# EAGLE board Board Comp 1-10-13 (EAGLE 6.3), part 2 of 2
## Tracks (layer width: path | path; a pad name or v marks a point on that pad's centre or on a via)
3.3V1  (via drill 0.61)
  Top 0.406: v91.72,21.72 107.04,21.72 108.41,20.34 109.17,20.34 SV1.6
  Bottom 0.406: 317CAP8.1 86.16,25.38 84.56,25.38 81.97,22.78 R7.1 81.81,22.55 81.81,21.49 80.52,20.19 80.52,18.21 80.82,17.91 84.63,17.91 88.75,22.02 IC4.4 88.9,22.1 89.28,21.72 v91.72,21.72
3.3V1_EN  (via drill 0.61)
  Top 0.406: v113.36,4.95 114.5,4.95 116.79,2.67 S1.19 | v101.62,6.4 98.65,6.4 98.27,6.02 96.37,6.02 v88.59,13.79
  Bottom 0.406: 317CAP3.1 93.17,56.46 93.17,52.2 91.95,50.98 80.82,50.98 79.15,49.3 79.15,16.76 80.82,15.09 85.7,15.09 86.54,15.93 IC4.3 86.61,15.77 v88.59,13.79 | v113.36,4.95 108.94,4.95 107.49,6.4 v101.62,6.4
3.3V1_EN1  (via drill 0.61)
  Top 0.406: v113.36,82.42 114.5,82.42 116.79,80.14 S2.19 | v101.62,83.87 98.65,83.87 98.27,83.49 96.37,83.49 v88.59,91.26
  Bottom 0.406: 317CAP1.1 93.17,133.93 93.17,129.67 91.95,128.45 80.82,128.45 79.15,126.77 79.15,94.23 80.82,92.56 85.7,92.56 86.54,93.4 IC3.3 86.61,93.24 v88.59,91.26 | v113.36,82.42 108.94,82.42 107.49,83.87 v101.62,83.87
3.3V2  (via drill 0.61)
  Top 0.406: v105.36,43.05 96.29,52.12 v91.72,52.12
  Bottom 0.406: 317CAP10.1 86.23,56.46 86.23,55.32 88.9,52.65 IC5.4 | R9.1 81.97,53.26 88.06,53.26 IC5.4 | v105.36,43.05 105.36,27.51 106.66,26.21 106.66,20.34 SV1.4 | v91.72,52.12 89.43,52.12 89.05,52.5 IC5.4
3.3V2_EN  (via drill 0.61)
  Top 0.406: v107.87,9.07 114.28,2.67 S1.18 | v97.05,33.3 v105.36,24.99
  Bottom 0.406: 92.63,43.13 91.34,43.13 89.97,41.76 88.06,41.76 87.53,42.29 87.53,45.49 IC5.3 | 92.63,43.13 93.78,43.13 317CAP9.1 | v107.87,9.07 107.87,14.86 105.36,17.37 v105.36,24.99 | v97.05,33.3 97.05,33.91 92.63,38.33 92.63,43.13
3.3V2_EN1  (via drill 0.61)
  Top 0.406: v107.87,86.54 114.28,80.14 S2.18 | v97.05,110.77 v105.36,102.46
  Bottom 0.406: 92.63,120.6 91.34,120.6 89.97,119.23 88.06,119.23 87.53,119.76 87.53,122.96 IC7.3 | 92.63,120.6 93.78,120.6 317CAP4.1 | v107.87,86.54 107.87,92.33 105.36,94.84 v105.36,102.46 | v97.05,110.77 97.05,111.38 92.63,115.8 92.63,120.6
3.3V3  (via drill 0.61)
  Top 0.406: v98.73,20.73 99.11,20.34 104.14,20.34 SV1.2
  Bottom 0.406: IC6.4 86.23,42.6 86.23,43.13 317CAP12.1 | IC6.4 | R11.1 81.97,39.93 88.67,39.93 IC6.4 | v98.73,20.73 98.73,30.02 88.98,39.78 IC6.4
3.3V3_EN  (via drill 0.61)
  Top 0.406: S1.17 111.76,3.12 105.36,9.53 100.79,9.53 90.73,19.58 90.73,24.23 v91.34,24.84
  Bottom 0.406: 93.17,26.52 93.17,27.66 92.33,28.5 92.33,35.05 92.02,35.36 88.14,35.36 86.54,33.76 IC6.3 | 93.17,26.52 93.17,25.45 317CAP11.1 | v91.34,24.84 93.02,26.52 93.17,26.52
3.3V3_EN1  (via drill 0.61)
  Top 0.406: S2.17 111.76,80.59 105.36,87 100.79,87 90.73,97.05 90.73,101.7 v91.34,102.31
  Bottom 0.406: 93.17,103.99 93.17,105.13 92.33,105.97 92.33,112.52 92.02,112.83 88.14,112.83 86.54,111.23 IC8.3 | 93.17,103.99 93.17,102.92 317CAP6.1 | v91.34,102.31 93.02,103.99 93.17,103.99
3.3V4  (via drill 0.61)
  Top 0.406: v98.73,98.2 99.11,97.81 104.14,97.81 SV5.2
  Bottom 0.406: IC8.4 86.23,120.07 86.23,120.6 317CAP7.1 | IC8.4 | R13.1 81.97,117.4 88.67,117.4 IC8.4 | v98.73,98.2 98.73,107.49 88.98,117.25 IC8.4
3.3V5  (via drill 0.61)
  Top 0.406: v91.72,99.19 107.04,99.19 108.41,97.81 109.17,97.81 SV5.6
  Bottom 0.406: 317CAP2.1 86.16,102.84 84.56,102.84 81.97,100.25 R3.1 81.81,100.03 81.81,98.96 80.52,97.66 80.52,95.68 80.82,95.38 84.63,95.38 88.75,99.49 IC3.4 88.9,99.57 89.28,99.19 v91.72,99.19
3.3V6  (via drill 0.61)
  Top 0.406: v105.36,120.52 96.29,129.59 v91.72,129.59
  Bottom 0.406: 317CAP5.1 86.23,133.93 86.23,132.79 88.9,130.12 IC7.4 | R5.1 81.97,130.73 88.06,130.73 IC7.4 | v105.36,120.52 105.36,104.98 106.66,103.68 106.66,97.81 SV5.4 | v91.72,129.59 89.43,129.59 89.05,129.97 IC7.4
5V1  (via drill 0.61)
  Top 0.406: v123.19,26.67 127.46,26.67 139.88,39.09 v139.88,41.99
  Bottom 0.406: C4.1 148.41,52.12 148.41,52.35 146.43,54.33 140.56,54.33 140.34,54.1 140.34,47.47 141.17,46.63 141.17,43.51 PWR_1.2 141.17,43.28 v139.88,41.99 | v123.19,26.67 SV1.12
5V1_EN  (via drill 0.61)
  Top 0.406: v126.01,4.8 124.48,3.28 124.48,2.67 S1.22 | v130.66,4.95 130.66,8.84 131.34,9.53 v131.34,21.41
  Bottom 0.406: C3.1 148.41,44.42 147.5,43.51 145.82,43.51 PWR_1.1 145.59,43.43 143.69,43.43 131.34,31.09 v131.34,21.41 | v126.01,4.8 130.5,4.8 v130.66,4.95
5V1_EN1  (via drill 0.61)
  Top 0.406: v126.01,82.27 124.48,80.75 124.48,80.14 S2.22 | v130.66,82.42 130.66,86.31 131.34,87 v131.34,98.88
  Bottom 0.406: C9.1 148.41,121.89 147.5,120.98 145.82,120.98 PWR_4.1 145.59,120.9 143.69,120.9 131.34,108.56 v131.34,98.88 | v126.01,82.27 130.5,82.27 v130.66,82.42
5V2  (via drill 0.61)
  Top 0.406: v147.8,36.12 v143.84,32.16 | v134.85,23.09 117.86,23.09 115.11,20.34 114.35,20.34 SV1.10
  Bottom 0.406: v143.84,32.16 141.25,29.57 PWR_2.2 141.1,29.34 v134.85,23.09 | v147.8,36.12 147.8,37.49 148.41,38.1 C6.1
5V2_EN  (via drill 0.61)
  Top 0.406: v124.56,4.88 124.18,4.88 121.97,2.67 S1.21 | v132.1,3.66 135.15,3.66 146.89,15.39 v146.89,27.81
  Bottom 0.406: 146.77,31.2 147.42,31.85 149.86,31.85 151.23,30.48 C5.1 | 146.77,31.2 145.82,30.25 145.82,29.57 PWR_2.1 | v124.56,4.88 125.78,3.66 v132.1,3.66 | v146.89,27.81 146.89,31.09 146.77,31.2
5V2_EN1  (via drill 0.61)
  Top 0.406: v124.56,82.35 124.18,82.35 121.97,80.14 S2.21 | v132.1,81.13 135.15,81.13 146.89,92.86 v146.89,105.28
  Bottom 0.406: 146.77,108.67 147.42,109.32 149.86,109.32 151.23,107.95 C11.1 | 146.77,108.67 145.82,107.72 145.82,107.04 PWR_5.1 | v124.56,82.35 125.78,81.13 v132.1,81.13 | v146.89,105.28 146.89,108.56 146.77,108.67
5V3  (via drill 0.61)
  Top 0.406: v141.17,18.14 135.23,24.08 116.33,24.08 112.6,20.34 111.76,20.34 SV1.8
  Bottom 0.406: C7.1 148.41,24.08 148.41,21.26 142.7,15.54 141.25,15.54 PWR_3.2 141.17,15.7 v141.17,18.14
5V3_EN  (via drill 0.61)
  Top 0.406: v125.32,5.94 122.81,5.94 119.53,2.67 119.38,2.67 S1.20 | v133.02,5.94 136.07,5.94 v144.37,14.25
  Bottom 0.406: C8.1 148.41,16.46 147.5,15.54 145.82,15.54 PWR_3.1 145.59,15.47 v144.37,14.25 | v133.02,5.94 v125.32,5.94
5V3_EN1  (via drill 0.61)
  Top 0.406: v125.32,83.41 122.81,83.41 119.53,80.14 119.38,80.14 S2.20 | v133.02,83.41 136.07,83.41 v144.37,91.72
  Bottom 0.406: C14.1 148.41,93.93 147.5,93.02 145.82,93.02 PWR_6.1 145.59,92.94 v144.37,91.72 | v133.02,83.41 v125.32,83.41
5V4  (via drill 0.61)
  Top 0.406: v141.17,95.61 135.23,101.55 116.33,101.55 112.6,97.81 111.76,97.81 SV5.8
  Bottom 0.406: C13.1 148.41,101.55 148.41,98.73 142.7,93.02 141.25,93.02 PWR_6.2 141.17,93.17 v141.17,95.61
5V5  (via drill 0.61)
  Top 0.406: v147.8,113.59 v143.84,109.63 | v134.85,100.56 117.86,100.56 115.11,97.81 114.35,97.81 SV5.10
  Bottom 0.406: v143.84,109.63 141.25,107.04 PWR_5.2 141.1,106.81 v134.85,100.56 | v147.8,113.59 147.8,114.96 148.41,115.57 C12.1
5V6  (via drill 0.61)
  Top 0.406: v123.19,104.14 127.46,104.14 139.88,116.56 v139.88,119.46
  Bottom 0.406: C10.1 148.41,129.59 148.41,129.82 146.43,131.8 140.56,131.8 140.34,131.57 140.34,124.94 141.17,124.1 141.17,120.98 PWR_4.2 141.17,120.75 v139.88,119.46 | v123.19,104.14 SV5.12
5V7
  Top 0.406: UP_TIME1.3 170.18,61.98 168.66,63.5 168.66,89.15 IC11.8 IC11.4 168.91,104.14 IC12.3
12V  (via drill 0.61)
  Top 0.406: 198.37,139.19 198.37,139.32 201.93,142.88 203.07,142.88 204.47,141.48 POWER.2 | 198.37,139.19 198.37,137.16 C1.1 | J2.1 161.29,138.05 162.81,136.53 163.7,136.53 167.89,140.72 167.89,144.91 U$2.1 167.89,145.03 167,145.92 167,148.46 167.77,149.22 170.05,149.22 173.1,146.18 178.56,146.18 | 178.56,146.18 182.25,146.18 U$4.8 | IC1.3 182.88,131.7 184.02,132.84 v184.02,133.73 | 178.56,146.18 v178.56,139.19 | v196.34,139.19 198.37,139.19
  Bottom 0.406: v184.02,133.73 v178.56,139.19 v196.34,139.19
12V1  (via drill 0.61)
  Top 0.406: 208.79,100.58 208.66,100.58 205.1,104.14 205.1,105.28 206.5,106.68 POWER1.2 | 208.79,100.58 210.82,100.58 C2.1 | J1.1 209.93,63.5 211.46,65.02 211.46,65.91 207.26,70.1 203.07,70.1 U$6.1 202.95,70.1 202.06,69.22 199.52,69.22 198.75,69.98 198.75,72.26 201.8,75.31 201.8,80.77 | 201.8,80.77 201.8,84.45 U$8.8 | IC2.3 216.28,85.09 215.14,86.23 v214.25,86.23 | 201.8,80.77 v208.79,80.77 | v208.79,98.55 208.79,100.58
  Bottom 0.406: v214.25,86.23 v208.79,80.77 v208.79,98.55
12V1_EN
  Top 0.406: S1.24 129.59,2.67 129.59,8.76 130.66,9.83 130.66,18.44 127.53,21.57 123.19,21.57 121.97,20.34 SV1.16
12V1_EN1
  Top 0.406: S2.24 129.59,80.14 129.59,86.23 130.66,87.3 130.66,95.91 127.53,99.03 123.19,99.03 121.97,97.81 SV5.16
12V2
  Top 1.27: SV1.18 124.48,20.34 127,20.34 SV1.20 127.38,19.81 128.68,18.52 128.68,11.2 | S1.11 101.62,11.2 S1.12 | S1.11 | S1.11 106.66,11.2 | 106.66,11.2 S1.10 | 106.66,11.2 109.17,11.2 S1.9 109.86,11.2 S1.8 | S1.8 | S1.8 114.28,11.2 | 114.28,11.2 S1.7 | 114.28,11.2 116.79,11.2 S1.6 117.47,11.2 S1.5 | S1.5 | S1.5 121.89,11.2 | 121.89,11.2 S1.4 | 121.89,11.2 124.41,11.2 S1.3 125.09,11.2 S1.2 | S1.2 | S1.2 128.68,11.2 | 128.68,11.2 129.51,11.2 S1.1
  Bottom 1.27: 12V_INPUT.1 117.32,62.87 128.68,51.51 128.68,22.02 127,20.34 SV1.20
12V2_EN  (via drill 0.61)
  Top 0.406: v127,8.91 S1.23
  Bottom 0.406: v127,8.91 127,10.97 120.6,17.37 120.6,19.05 119.38,20.27 SV1.14
12V2_EN1  (via drill 0.61)
  Top 0.406: v127,86.39 S2.23
  Bottom 0.406: v127,86.39 127,88.44 120.6,94.84 120.6,96.52 119.38,97.74 SV5.14
12V3
  Top 1.27: SV5.18 124.48,97.81 127,97.81 SV5.20 127.38,97.28 128.68,95.99 128.68,88.67 | S2.11 101.62,88.67 S2.12 | S2.11 | S2.11 106.66,88.67 | 106.66,88.67 S2.10 | 106.66,88.67 109.17,88.67 S2.9 109.86,88.67 S2.8 | S2.8 | S2.8 114.28,88.67 | 114.28,88.67 S2.7 | 114.28,88.67 116.79,88.67 S2.6 117.47,88.67 S2.5 | S2.5 | S2.5 121.89,88.67 | 121.89,88.67 S2.4 | 121.89,88.67 124.41,88.67 S2.3 125.09,88.67 S2.2 | S2.2 | S2.2 128.68,88.67 | 128.68,88.67 129.51,88.67 S2.1
  Bottom 1.27: 12V_INPUT1.1 117.32,140.34 128.68,128.98 128.68,99.49 127,97.81 SV5.20
12V4
  Top 2.54: 72.39,100.84 R15.2 R16.2 67.31,100.84 66.24,101.55 64.29,103.5 55.78,103.5 53.82,105.46 53.82,122.15 54.71,123.04 | 54.71,123.04 54.86,122.89 56.84,122.89 D3.C | 54.71,123.04 52.93,124.82 45.59,124.82 44.35,123.57 44.35,123.55 44.12,123.32 44.12,123.14 43.99,123.01 43.99,122.89 43.28,122.17 43.28,122 41.94,120.65 K2.P1
12V5
  Top 2.54: 72.39,23.37 R21.2 R22.2 67.31,23.37 66.24,24.08 64.29,26.04 55.78,26.04 53.82,27.99 53.82,44.68 54.71,45.57 | 54.71,45.57 54.86,45.41 56.84,45.41 D1.C | 54.71,45.57 52.93,47.35 45.59,47.35 44.35,46.1 44.35,46.08 44.12,45.85 44.12,45.67 43.99,45.54 43.99,45.41 43.28,44.7 43.28,44.53 41.94,43.18 K4.P1
12V6  (via drill 0.61)
  Top 0.406: 208.79,43.43 208.66,43.43 205.1,46.99 205.1,48.13 206.5,49.53 POWER4.2 | 208.79,43.43 210.82,43.43 C21.1 | J3.1 209.93,6.35 211.46,7.87 211.46,8.76 207.26,12.95 203.07,12.95 U$12.1 202.95,12.95 202.06,12.06 199.52,12.06 198.75,12.83 198.75,15.11 201.8,18.16 201.8,23.62 | 201.8,23.62 201.8,27.3 U$14.8 | IC13.3 216.28,27.94 215.14,29.08 v214.25,29.08 | 201.8,23.62 v208.79,23.62 | v208.79,41.4 208.79,43.43
  Bottom 0.406: v214.25,29.08 v208.79,23.62 v208.79,41.4
12V7  (via drill 0.61)
  Top 0.406: 235.46,100.58 235.33,100.58 231.78,104.14 231.78,105.28 233.17,106.68 POWER5.2 | 235.46,100.58 237.49,100.58 C15.1 | J4.1 236.6,63.5 238.12,65.02 238.12,65.91 233.93,70.1 229.74,70.1 U$16.1 229.62,70.1 228.73,69.22 226.19,69.22 225.43,69.98 225.43,72.26 228.47,75.31 228.47,80.77 | 228.47,80.77 228.47,84.45 U$18.8 | IC9.3 242.95,85.09 241.81,86.23 v240.92,86.23 | 228.47,80.77 v235.46,80.77 | v235.46,98.55 235.46,100.58
  Bottom 0.406: v240.92,86.23 v235.46,80.77 v235.46,98.55
12V8  (via drill 0.61)
  Top 0.406: 235.46,43.43 235.33,43.43 231.78,46.99 231.78,48.13 233.17,49.53 POWER6.2 | 235.46,43.43 237.49,43.43 C16.1 | J5.1 236.6,6.35 238.12,7.87 238.12,8.76 233.93,12.95 229.74,12.95 U$20.1 229.62,12.95 228.73,12.06 226.19,12.06 225.43,12.83 225.43,15.11 228.47,18.16 228.47,23.62 | 228.47,23.62 228.47,27.3 U$22.8 | IC10.3 242.95,27.94 241.81,29.08 v240.92,29.08 | 228.47,23.62 v235.46,23.62 | v235.46,41.4 235.46,43.43
  Bottom 0.406: v240.92,29.08 v235.46,23.62 v235.46,41.4
12V_PRE
  Top 2.54: D3.A 65.02,107.95 69.47,112.39 POWER2.2
12V_PRE1
  Top 2.54: D1.A 65.02,30.48 69.47,34.92 POWER3.2
24V1
  Top 0.406: IC12.1 177.8,106.68 C20.+ | LED9.A 162.69,35.56 173.99,24.26 X2.3
  Bottom 0.406: C20.+ 184.15,106.81 186.94,104.01 186.94,62.48 LED9.A
DIR
  Top 0.406: R17.2 53.34,146.51 51.61,148.23 51.05,148.23 IO.2
DIR1
  Top 0.406: R23.2 53.34,69.04 51.61,70.76 51.05,70.76 IO1.2
GND
  pour Top: 156.21,152.4 156.21,129.54 209.55,129.54 209.55,152.4
  pour Bottom: 156.21,152.4 156.21,129.54 209.55,129.54 209.55,152.4
GND1
  pour Top: 195.58,58.42 218.44,58.42 218.44,111.76 195.58,111.76
  pour Bottom: 195.58,58.42 218.44,58.42 218.44,111.76 195.58,111.76
GND2  (via drill 0.61)
  Top 0.406: U$9.9 137.52,67.28 137.52,62.26 U$9.7 137.36,62.18 136.6,62.18 134.43,60.01 | SV4.1 104.14,48.31 106.66,48.31 SV4.3 106.88,48.23 109.17,48.23 SV4.5 109.4,48.31 111.76,48.31 SV4.7 111.91,48.31 114.28,48.31 SV4.9 114.5,48.23 116.79,48.23 SV4.11 117.02,48.31 119.38,48.31 SV4.13 119.53,48.31 121.89,48.31 SV4.15 122.12,48.23 124.41,48.23 SV4.17 124.64,48.31 125.78,48.31 | 125.78,48.31 127,48.31 SV4.19 127.08,48.08 127.08,42.29 128.22,41.15 128.22,39.4 127.08,38.25 SV3.19 SV3.17 SV3.15 SV3.13 SV3.11 SV3.9 SV3.7 SV3.5 SV3.3 SV3.1 104.06,37.95 104.06,32.16 102.92,31.01 102.92,29.26 104.06,28.12 SV2.1 104.14,27.96 106.66,27.96 SV2.3 106.81,27.96 109.17,27.96 SV2.5 109.4,27.96 110.54,27.96 | 134.43,60.01 125.78,51.36 125.78,48.31 | SV1.1 104.14,17.83 106.66,17.83 SV1.3 | 110.54,27.96 111.76,27.96 SV2.7 111.91,27.96 114.28,27.96 SV2.9 114.43,27.96 116.79,27.96 SV2.11 117.02,27.96 119.38,27.96 SV2.13 119.53,27.96 121.89,27.96 SV2.15 122.05,27.96 124.41,27.96 SV2.17 124.64,27.96 127,27.96 SV2.19 | SV1.19 127,17.83 124.64,17.83 SV1.17 124.41,17.83 121.97,17.83 SV1.15 121.74,17.83 119.38,17.83 SV1.13 | 110.54,19.05 110.54,27.96 | 110.54,19.05 111.76,17.83 SV1.7 | SV1.5 109.25,17.83 110.39,18.97 110.54,19.05 | 134.43,60.01 v130.89,63.55
  Bottom 0.406: 130.66,63.55 130.66,65.99 V7805_C5.2 130.66,66.22 130.66,69.19 | 130.66,63.55 130.66,61.65 V7805_C6.2 | 130.66,69.19 130.66,70.48 V7805_C4.2 | 130.66,69.19 116.86,69.19 12V_INPUT.2 116.71,69.19 101.78,69.19 TS7800_CON.2 | R12.2 81.89,36.35 81.89,36.5 79.83,38.56 79.83,47.55 81.89,49.61 R10.2 | SV1.3 106.73,17.75 108.94,17.75 SV1.5 | C6.2 151.23,38.1 151.23,44.42 C3.2 | SV1.7 111.76,17.83 114.12,17.83 SV1.9 114.58,17.75 116.79,17.75 SV1.11 117.02,17.83 119.38,17.83 SV1.13 | v130.89,63.55 130.66,63.55
  pour Top: 78.74,74.93 152.4,74.93 152.4,1.27 78.74,1.27
  pour Bottom: 78.74,74.93 152.4,74.93 152.4,1.27 78.74,1.27
GND3  (via drill 0.61)
  Top 0.406: U$10.9 137.52,144.75 137.52,139.72 U$10.7 137.36,139.65 136.6,139.65 134.43,137.48 | SV8.1 104.14,125.78 106.66,125.78 SV8.3 106.88,125.7 109.17,125.7 SV8.5 109.4,125.78 111.76,125.78 SV8.7 111.91,125.78 114.28,125.78 SV8.9 114.5,125.7 116.79,125.7 SV8.11 117.02,125.78 119.38,125.78 SV8.13 119.53,125.78 121.89,125.78 SV8.15 122.12,125.7 124.41,125.7 SV8.17 124.64,125.78 125.78,125.78 | 125.78,125.78 127,125.78 SV8.19 127.08,125.55 127.08,119.76 128.22,118.62 128.22,116.86 127.08,115.72 SV7.19 SV7.17 SV7.15 SV7.13 SV7.11 SV7.9 SV7.7 SV7.5 SV7.3 SV7.1 104.06,115.42 104.06,109.63 102.92,108.48 102.92,106.73 104.06,105.59 SV6.1 104.14,105.44 106.66,105.44 SV6.3 106.81,105.44 109.17,105.44 SV6.5 109.4,105.44 110.54,105.44 | 134.43,137.48 125.78,128.83 125.78,125.78 | SV5.1 104.14,95.3 106.66,95.3 SV5.3 | 110.54,105.44 111.76,105.44 SV6.7 111.91,105.44 114.28,105.44 SV6.9 114.43,105.44 116.79,105.44 SV6.11 117.02,105.44 119.38,105.44 SV6.13 119.53,105.44 121.89,105.44 SV6.15 122.05,105.44 124.41,105.44 SV6.17 124.64,105.44 127,105.44 SV6.19 | SV5.19 127,95.3 124.64,95.3 SV5.17 124.41,95.3 121.97,95.3 SV5.15 121.74,95.3 119.38,95.3 SV5.13 | 110.54,96.52 110.54,105.44 | 110.54,96.52 111.76,95.3 SV5.7 | SV5.5 109.25,95.3 110.39,96.44 110.54,96.52 | 134.43,137.48 v130.89,141.02
  Bottom 0.406: 130.66,141.02 130.66,143.46 V7805_C2.2 130.66,143.69 130.66,146.66 | 130.66,141.02 130.66,139.12 V7805_C3.2 | 130.66,146.66 130.66,147.96 V7805_C1.2 | 130.66,146.66 116.86,146.66 12V_INPUT1.2 116.71,146.66 101.78,146.66 TS7800_CON1.2 | R14.2 81.89,113.82 81.89,113.97 79.83,116.03 79.83,125.02 81.89,127.08 R6.2 | SV5.3 106.73,95.22 108.94,95.22 SV5.5 | C12.2 151.23,115.57 151.23,121.89 C9.2 | SV5.7 111.76,95.3 114.12,95.3 SV5.9 114.58,95.22 116.79,95.22 SV5.11 117.02,95.3 119.38,95.3 SV5.13 | v130.89,141.02 130.66,141.02
  pour Top: 78.74,152.4 152.4,152.4 152.4,78.74 78.74,78.74
  pour Bottom: 78.74,152.4 152.4,152.4 152.4,78.74 78.74,78.74
GND4
  pour Top: 222.25,58.42 245.11,58.42 245.11,111.76 222.25,111.76
  pour Bottom: 222.25,58.42 245.11,58.42 245.11,111.76 222.25,111.76
GND5
  pour Bottom: 156.21,1.27 191.77,1.27 191.77,125.73 156.21,125.73
  pour Top: 156.21,1.27 191.77,1.27 191.77,125.73 156.21,125.73
GND6
  pour Top: 1.27,152.4 74.93,152.4 74.93,78.74 1.27,78.74
  pour Bottom: 1.27,152.4 74.93,152.4 74.93,78.74 1.27,78.74
GND7
  pour Top: 1.27,74.93 74.93,74.93 74.93,1.27 1.27,1.27
  pour Bottom: 1.27,74.93 74.93,74.93 74.93,1.27 1.27,1.27
GND8
  pour Top: 195.58,1.27 218.44,1.27 218.44,54.61 195.58,54.61
  pour Bottom: 195.58,1.27 218.44,1.27 218.44,54.61 195.58,54.61
GND9
  pour Top: 222.25,1.27 245.11,1.27 245.11,54.61 222.25,54.61
  pour Bottom: 222.25,1.27 245.11,1.27 245.11,54.61 222.25,54.61
MOTOR+
  Bottom 2.54: K1.O2 36.96,97.92 38.23,99.19 38.23,99.67 39.22,100.66 39.22,100.71 40.18,101.68 40.31,101.68 40.49,101.85 40.77,101.85 40.89,101.98 41.02,101.98 41.1,101.91 43.31,101.91 43.59,101.62 43.66,101.7 43.71,101.7 44.91,102.89 44.91,103.35 46.91,105.36 46.91,105.41 K1.S1 47.98,106.15 50.11,108.28 50.11,124.28 27.66,146.74 27.66,147.32 OUTPUT.2
MOTOR+1
  Bottom 2.54: K3.O2 36.96,20.45 38.23,21.72 38.23,22.2 39.22,23.19 39.22,23.24 40.18,24.21 40.31,24.21 40.49,24.38 40.77,24.38 40.89,24.51 41.02,24.51 41.1,24.43 43.31,24.43 43.59,24.16 43.66,24.23 43.71,24.23 44.91,25.43 44.91,25.88 46.91,27.89 46.91,27.94 K3.S1 47.98,28.68 50.11,30.81 50.11,46.81 27.66,69.27 27.66,69.85 OUTPUT1.2
MOTOR-
  Top 2.54: K1.S2 46.91,97.92 46.91,97.97 44.91,99.97 44.91,100.43 43.71,101.62 43.66,101.62 43.59,101.7 43.31,101.42 41.1,101.42 41.02,101.35 40.89,101.35 40.77,101.47 40.49,101.47 40.31,101.65 40.18,101.65 39.22,102.62 39.22,102.67 38.23,103.66 38.23,104.14 36.96,105.41 K1.O1 35.89,106.15 34.14,107.9 34.14,133.91 21.31,146.74 OUTPUT.1
MOTOR-1
  Top 2.54: K3.S2 46.91,20.45 46.91,20.5 44.91,22.5 44.91,22.96 43.71,24.16 43.66,24.16 43.59,24.23 43.31,23.95 41.1,23.95 41.02,23.88 40.89,23.88 40.77,24 40.49,24 40.31,24.18 40.18,24.18 39.22,25.15 39.22,25.2 38.23,26.19 38.23,26.67 36.96,27.94 K3.O1 35.89,28.68 34.14,30.43 34.14,56.44 21.31,69.27 OUTPUT1.1
N$1  (via drill 0.61)
  Top 0.406: v189.48,132.08 U$1.1 | v182.75,132.97 181.61,131.83 IC1.2
  Bottom 0.406: v189.48,132.08 183.64,132.08 v182.75,132.97
N$2  (via drill 0.61)
  Top 0.406: v198.37,135.13 198.37,132.08 U$1.2 | v198.37,141.99 200.03,143.64 U$3.1
  Bottom 0.406: v198.37,141.99 v198.37,135.13
N$3  (via drill 0.61)
  Top 0.406: IC1.4 184.15,131.95 v185.29,133.1 | v180.97,138.18 178.05,138.18 171.07,131.19 168.91,131.19 R1.2
  Bottom 0.406: v185.29,133.1 185.29,133.86 v180.97,138.18
N$4
  Top 0.406: U$2.2 169.8,144.91 169.8,139.19 166.24,135.64 R1.3
N$5
  Top 0.406: C1.2 195.33,137.16 195.33,144.4 193.68,146.05 U$3.4 | U$3.4 U$3.2 | J2.2 161.29,143.76 167.51,149.99 189.48,149.99 193.55,145.92 U$3.4
N$6  (via drill 0.61)
  Top 0.406: v215.9,91.69 U$5.1 | v215.01,84.96 216.15,83.82 IC2.2
  Bottom 0.406: v215.9,91.69 215.9,85.85 v215.01,84.96
N$7  (via drill 0.61)
  Top 0.406: IC2.4 216.03,86.36 v214.88,87.5 | v209.8,83.19 209.8,80.26 216.79,73.28 216.79,71.12 R2.2
  Bottom 0.406: v214.88,87.5 214.12,87.5 v209.8,83.19
N$8
  Top 0.406: IC1.5 185.42,131.57 187.58,133.73 188.72,133.73 189.48,134.49 189.48,136.53 187.58,138.43 183.9,138.43 182.25,140.08 U$4.1
N$9
  Top 0.406: U$6.2 203.07,72.01 208.79,72.01 212.34,68.45 R2.3
N$10  (via drill 0.61)
  Top 0.406: v212.85,100.58 215.9,100.58 U$5.2 | v205.99,100.58 204.34,102.23 U$7.1
  Bottom 0.406: v205.99,100.58 v212.85,100.58
N$11
  Top 0.406: C2.2 210.82,97.54 203.58,97.54 201.93,95.89 U$7.4 | U$7.4 U$7.2 | J1.2 204.22,63.5 197.99,69.72 197.99,91.69 202.06,95.76 U$7.4
N$12
  Top 0.406: IC2.5 216.41,87.63 214.25,89.79 214.25,90.93 213.49,91.69 211.46,91.69 209.55,89.79 209.55,86.11 207.9,84.45 U$8.1
N$13
  Bottom 0.406: IC4.1 91.26,16 89.74,17.53 85.78,17.53 84.63,16.38 81.97,16.38 R8.1 81.74,16.46 81.28,16.46 79.83,17.91 79.83,23.01 81.89,25.07 81.89,25.53 R7.2
N$14  (via drill 0.61)
  Top 0.406: v83.87,47.02 v83.87,56.01
  Bottom 0.406: 83.87,46.86 84.63,46.86 85.78,48.01 89.74,48.01 91.26,46.48 IC5.1 | 83.87,46.86 81.97,46.86 R10.1 | v83.87,56.01 81.97,56.01 R9.2 | v83.87,47.02 83.87,46.86
N$15
  Bottom 0.406: 83.34,33.45 84.48,33.45 85.78,32.16 89.74,32.16 91.26,33.68 IC6.1 | 83.34,33.45 81.97,33.45 R12.1 | 83.34,33.45 83.34,37.34 83.03,37.64 81.74,37.64 80.52,38.86 80.52,40.84 81.89,42.22 81.89,42.67 R11.2
N$16  (via drill 0.61)
  Top 0.406: v138.89,65.15 138.89,61.04 137.59,59.74 U$9.6
  Bottom 0.406: v138.89,65.15 133.55,70.48 V7805_C4.1
N$17
  Bottom 0.406: IC3.1 91.26,93.47 89.74,95 85.78,95 84.63,93.85 81.97,93.85 R4.1 81.74,93.93 81.28,93.93 79.83,95.38 79.83,100.48 81.89,102.54 81.89,103 R3.2
N$18  (via drill 0.61)
  Top 0.406: v83.87,124.48 v83.87,133.48
  Bottom 0.406: 83.87,124.33 84.63,124.33 85.78,125.48 89.74,125.48 91.26,123.95 IC7.1 | 83.87,124.33 81.97,124.33 R6.1 | v83.87,133.48 81.97,133.48 R5.2 | v83.87,124.48 83.87,124.33
N$19
  Bottom 0.406: 83.34,110.92 84.48,110.92 85.78,109.63 89.74,109.63 91.26,111.15 IC8.1 | 83.34,110.92 81.97,110.92 R14.1 | 83.34,110.92 83.34,114.81 83.03,115.11 81.74,115.11 80.52,116.33 80.52,118.31 81.89,119.69 81.89,120.14 R13.2
N$20  (via drill 0.61)
  Top 0.406: v138.89,142.62 138.89,138.51 137.59,137.21 U$10.6
  Bottom 0.406: v138.89,142.62 133.55,147.96 V7805_C1.1
N$21  (via drill 0.61)
  Top 0.406: v242.57,91.69 U$15.1 | v241.68,84.96 242.82,83.82 IC9.2
  Bottom 0.406: v242.57,91.69 242.57,85.85 v241.68,84.96
N$22  (via drill 0.61)
  Top 0.406: IC9.4 242.7,86.36 v241.55,87.5 | v236.47,83.19 236.47,80.26 243.46,73.28 243.46,71.12 R28.2
  Bottom 0.406: v241.55,87.5 240.79,87.5 v236.47,83.19
N$23
  Top 0.406: U$16.2 229.74,72.01 235.46,72.01 239.01,68.45 R28.3
N$24  (via drill 0.61)
  Top 0.406: v239.52,100.58 242.57,100.58 U$15.2 | v232.66,100.58 231.01,102.23 U$17.1
  Bottom 0.406: v232.66,100.58 v239.52,100.58
N$25
  Top 0.406: C15.2 237.49,97.54 230.25,97.54 228.6,95.89 U$17.4 | U$17.4 U$17.2 | J4.2 230.89,63.5 224.66,69.72 224.66,91.69 228.73,95.76 U$17.4
N$26
  Top 0.406: IC9.5 243.08,87.63 240.92,89.79 240.92,90.93 240.16,91.69 238.12,91.69 236.22,89.79 236.22,86.11 234.57,84.45 U$18.1
N$27  (via drill 0.61)
  Top 0.406: v242.57,34.54 U$19.1 | v241.68,27.81 242.82,26.67 IC10.2
  Bottom 0.406: v242.57,34.54 242.57,28.7 v241.68,27.81
N$28  (via drill 0.61)
  Top 0.406: IC10.4 242.7,29.21 v241.55,30.35 | v236.47,26.04 236.47,23.11 243.46,16.13 243.46,13.97 R29.2
  Bottom 0.406: v241.55,30.35 240.79,30.35 v236.47,26.04
N$29
  Top 0.406: U$20.2 229.74,14.86 235.46,14.86 239.01,11.3 R29.3
N$30  (via drill 0.61)
  Top 0.406: v239.52,43.43 242.57,43.43 U$19.2 | v232.66,43.43 231.01,45.09 U$21.1
  Bottom 0.406: v232.66,43.43 v239.52,43.43
N$31
  Top 0.406: C16.2 237.49,40.39 230.25,40.39 228.6,38.73 U$21.4 | U$21.4 U$21.2 | J5.2 230.89,6.35 224.66,12.57 224.66,34.54 228.73,38.61 U$21.4
N$32
  Top 0.406: IC10.5 243.08,30.48 240.92,32.64 240.92,33.78 240.16,34.54 238.12,34.54 236.22,32.64 236.22,28.96 234.57,27.3 U$22.1
N$34
  Top 0.406: IC11.2 175.26,92.46 186.18,81.53 186.18,37.59 C18.+
  Bottom 0.406: IC11.2 170.18,92.71 IC11.6
N$35
  Top 0.406: IC11.5 167.64,97.54 165.1,95 165.1,48.26 DOWN_TIME1.2
  Bottom 0.406: DOWN_TIME1.2 167.64,54.36 184.15,70.87 C19.+
N$36
  Top 0.406: DOWN_TIME1.3 170.18,46.74 167.64,49.28 UP_TIME1.2 165.86,62.74 165.86,90.68 167.64,92.46 IC11.7
N$37
  Top 0.406: LED10.A LED9.K
N$38
  Top 0.406: LED11.A LED10.K
N$39
  Top 0.406: LED12.A LED11.K
N$40
  Top 0.406: LED13.A LED12.K
N$41
  Top 0.406: LED15.A LED13.K
N$42
  Top 0.406: LED14.A LED15.K
N$43
  Top 0.406: LED16.A LED14.K
N$44
  Bottom 0.406: BRIGHTNESS1.2 167.64,87.88 161.16,94.36 161.16,116.97 LED16.K
N$45
  Bottom 0.406: BRIGHTNESS1.3 170.18,78.49 186.18,94.49 186.18,103.76 170.56,119.38 Q2.D
N$46
  Bottom 0.406: IC11.3 175.26,95.5 167.64,103.12 167.64,119.38 Q2.G
N$47
  Top 2.54: K2.S1 47.24,120.65 50.11,117.78 50.11,95.61 48.26,93.75 45.59,93.75 44.35,95 44.35,95.02 43.2,96.16 43.2,96.65 41.94,97.92 K1.P2
N$48
  Top 2.54: K1.P1 41.94,105.41 43.2,106.68 43.2,107.16 44.35,108.31 44.35,108.33 44.63,108.61 44.63,110.01 44.91,110.29 44.91,110.44 45.49,111.02 45.49,111.73 46.91,113.16 K2.S2
N$49
  Top 0.406: R15.1 72.39,97.99 70.61,97.99 63.98,91.36 29.59,91.36 23.65,97.31 22.55,97.31 21.95,97.92 K1.1
N$50
  Top 0.406: R16.1 67.31,97.99 54.97,97.99 49,92.02 43.84,92.02 39.06,96.8 39.06,99.77 36.52,102.31 33.88,102.31 23.65,112.55 22.55,112.55 21.95,113.16 K2.1
N$51
  Top 0.406: T1.3 15.09,105.08 21.59,105.08 K1.2
N$52
  Top 0.406: T2.3 15.09,120.32 21.59,120.32 K2.2
N$53  (via drill 0.61)
  Top 0.406: v14.38,122.4 13.23,121.26 T2.1 | v41.5,130 44.73,133.22 45.74,133.22 46.08,133.55 46.35,133.55 R18.1
  Bottom 0.406: v14.38,122.4 19.71,122.4 27.3,130 v41.5,130
N$54  (via drill 0.61)
  Top 0.406: v14.38,107.16 13.23,106.02 T1.1 | v42.11,123.9 42.22,123.9 51.54,133.22 52.73,133.22 53.06,133.55 53.34,133.55 R17.1
  Bottom 0.406: v14.38,107.16 19.71,107.16 22.78,110.24 27.53,110.24 41.2,123.9 v42.11,123.9
N$55  (via drill 0.61)
  Top 0.406: v22.81,102.31 15.04,102.31 13.23,104.11 T1.2 | v39.8,119.3 39.8,123.01 v50.01,133.22 | v64.44,133.22 65.68,134.47 66.73,134.47 67.03,134.77 R19.2 | R19.2
  Bottom 0.406: v39.8,119.3 v22.81,102.31 | v64.44,133.22 v50.01,133.22
N$56  (via drill 0.61)
  Top 0.406: v27.64,117.55 15.04,117.55 13.23,119.36 T2.2 | v44.27,134.19 v39.12,129.03 | v70.46,134.19 70.74,134.47 71.81,134.47 72.11,134.77 R20.2 | R20.2
  Bottom 0.406: v39.12,129.03 v27.64,117.55 | v70.46,134.19 v44.27,134.19
N$57
  Top 2.54: K4.S1 47.24,43.18 50.11,40.31 50.11,18.14 48.26,16.28 45.59,16.28 44.35,17.53 44.35,17.55 43.2,18.69 43.2,19.18 41.94,20.45 K3.P2
N$58
  Top 2.54: K3.P1 41.94,27.94 43.2,29.21 43.2,29.69 44.35,30.84 44.35,30.86 44.63,31.14 44.63,32.54 44.91,32.82 44.91,32.97 45.49,33.55 45.49,34.27 46.91,35.69 K4.S2
N$59
  Top 0.406: R21.1 72.39,20.52 70.61,20.52 63.98,13.89 29.59,13.89 23.65,19.84 22.55,19.84 21.95,20.45 K3.1
N$60
  Top 0.406: R22.1 67.31,20.52 54.97,20.52 49,14.55 43.84,14.55 39.06,19.33 39.06,22.3 36.52,24.84 33.88,24.84 23.65,35.08 22.55,35.08 21.95,35.69 K4.1
N$61
  Top 0.406: T3.3 15.09,27.61 21.59,27.61 K3.2
N$62
  Top 0.406: T4.3 15.09,42.85 21.59,42.85 K4.2
N$63  (via drill 0.61)
  Top 0.406: v14.38,44.93 13.23,43.79 T4.1 | v41.5,52.53 44.73,55.75 45.74,55.75 46.08,56.08 46.35,56.08 R24.1
  Bottom 0.406: v14.38,44.93 19.71,44.93 27.3,52.53 v41.5,52.53
N$64  (via drill 0.61)
  Top 0.406: v14.38,29.69 13.23,28.55 T3.1 | v42.11,46.43 42.22,46.43 51.54,55.75 52.73,55.75 53.06,56.08 53.34,56.08 R23.1
  Bottom 0.406: v14.38,29.69 19.71,29.69 22.78,32.77 27.53,32.77 41.2,46.43 v42.11,46.43
N$65  (via drill 0.61)
  Top 0.406: v22.81,24.84 15.04,24.84 13.23,26.64 T3.2 | v39.8,41.83 39.8,45.54 v50.01,55.75 | v64.44,55.75 65.68,57 66.73,57 67.03,57.3 R25.2 | R25.2
  Bottom 0.406: v39.8,41.83 v22.81,24.84 | v64.44,55.75 v50.01,55.75
N$66  (via drill 0.61)
  Top 0.406: v27.64,40.08 15.04,40.08 13.23,41.88 T4.2 | v44.27,56.72 v39.12,51.56 | v70.46,56.72 70.74,57 71.81,57 72.11,57.3 R26.2 | R26.2
  Bottom 0.406: v39.12,51.56 v27.64,40.08 | v70.46,56.72 v44.27,56.72
N$67  (via drill 0.61)
  Top 0.406: v215.9,34.54 U$11.1 | v215.01,27.81 216.15,26.67 IC13.2
  Bottom 0.406: v215.9,34.54 215.9,28.7 v215.01,27.81
N$68  (via drill 0.61)
  Top 0.406: IC13.4 216.03,29.21 v214.88,30.35 | v209.8,26.04 209.8,23.11 216.79,16.13 216.79,13.97 R27.2
  Bottom 0.406: v214.88,30.35 214.12,30.35 v209.8,26.04
N$69
  Top 0.406: U$12.2 203.07,14.86 208.79,14.86 212.34,11.3 R27.3
N$70  (via drill 0.61)
  Top 0.406: v212.85,43.43 215.9,43.43 U$11.2 | v205.99,43.43 204.34,45.09 U$13.1
  Bottom 0.406: v205.99,43.43 v212.85,43.43
N$71
  Top 0.406: C21.2 210.82,40.39 203.58,40.39 201.93,38.73 U$13.4 | U$13.4 U$13.2 | J3.2 204.22,6.35 197.99,12.57 197.99,34.54 202.06,38.61 U$13.4
N$72
  Top 0.406: IC13.5 216.41,30.48 214.25,32.64 214.25,33.78 213.49,34.54 211.46,34.54 209.55,32.64 209.55,28.96 207.9,27.3 U$14.1
ON
  Top 0.406: R18.2 46.35,147.14 47.45,148.23 48.01,148.23 IO.1
ON1
  Top 0.406: R24.2 46.35,69.67 47.45,70.76 48.01,70.76 IO1.1
TS7800_+  (via drill 0.89)
  Top 1.27: v128.75,59.74 126.69,59.74 U$9.5 126.01,59.82 104.67,59.82 101.62,62.87 TS7800_CON.1
  Bottom 1.27: v128.75,59.74 131.8,59.74 133.48,61.42 133.48,61.57 V7805_C6.1
TS7800_+1  (via drill 0.89)
  Top 1.27: v128.75,137.21 126.69,137.21 U$10.5 126.01,137.29 104.67,137.29 101.62,140.34 TS7800_CON1.1
  Bottom 1.27: v128.75,137.21 131.8,137.21 133.48,138.89 133.48,139.04 V7805_C3.1
TS7800_EN  (via drill 0.89)
  Top 1.27: v131.8,68.2 128.29,68.2 126.69,69.8 U$9.1 126.16,69.42 123.11,66.37 101.09,66.37 87.15,52.43 87.15,8.46 93.93,1.68 99.87,1.68 100.79,2.59 101.55,2.59 S1.13
  Bottom 1.27: v131.8,68.2 133.48,66.52 133.48,66.06 V7805_C5.1
TS7800_EN1  (via drill 0.89)
  Top 1.27: v131.8,145.67 128.29,145.67 126.69,147.27 U$10.1 126.16,146.89 123.11,143.84 101.09,143.84 87.15,129.9 87.15,85.93 93.93,79.15 99.87,79.15 100.79,80.06 101.55,80.06 S2.13
  Bottom 1.27: v131.8,145.67 133.48,143.99 133.48,143.53 V7805_C2.1
VREF1  (via drill 0.61)
  Top 0.406: SV3.20 127,40.69 124.64,40.69 SV3.18 124.41,40.62 122.12,40.62 SV3.16 121.89,40.69 119.53,40.69 SV3.14 119.38,40.69 117.02,40.69 SV3.12 116.79,40.62 114.5,40.62 SV3.10 114.28,40.69 111.91,40.69 SV3.8 111.76,40.69 109.4,40.69 SV3.6 109.17,40.62 106.88,40.62 SV3.4 106.66,40.69 104.14,40.69 SV3.2 103.99,40.54 102.92,40.54 90.04,27.66 90.04,14.86 v97.89,7.01
  Bottom 0.406: 97.78,6.06 100.56,3.28 114.58,3.28 118.01,6.71 118.01,7.62 119.38,8.99 6103CAP8.1 | 97.78,6.06 97.66,6.17 96.22,6.17 3V3.2 | v97.89,7.01 97.89,6.17 97.78,6.06
VREF1_EN  (via drill 0.61)
  Top 0.406: v105.44,8.08 105.82,8.08 109.17,4.72 109.17,2.67 S1.16 | v132.94,4.65 132.03,5.56 132.03,20.73 132.33,21.03 132.33,21.79 131.72,22.4 119.69,22.4 118.08,20.8 118.08,17.3 114.28,13.49 v106.88,13.49
  Bottom 0.406: 3V3.1 96.22,8.08 v105.44,8.08 105.51,8.23 106.88,9.6 v106.88,13.49 | v132.94,4.65 134.47,3.12 134.47,2.59 6103CAP7.1
VREF1_EN1  (via drill 0.61)
  Top 0.406: v105.44,85.55 105.82,85.55 109.17,82.19 109.17,80.14 S2.16 | v132.94,82.12 132.03,83.03 132.03,98.2 132.33,98.5 132.33,99.26 131.72,99.87 119.69,99.87 118.08,98.27 118.08,94.77 114.28,90.96 v106.88,90.96
  Bottom 0.406: 3V1.1 96.22,85.55 v105.44,85.55 105.51,85.7 106.88,87.07 v106.88,90.96 | v132.94,82.12 134.47,80.59 134.47,80.06 6103CAP1.1
VREF2
  Top 0.406: SV2.2 SV2.4 SV2.6 SV2.8 SV2.10 SV2.12 SV2.14 SV2.16 SV2.18 SV2.20
  Bottom 0.406: 3V4.2 114.12,6.71 112.83,6.71 110.54,8.99 6103CAP10.1 110.54,9.22 110.54,29.26 SV2.8
VREF2_EN  (via drill 0.61)
  Top 0.406: v107.95,4.57 107.95,3.89 106.73,2.67 S1.15 | v94.08,4.5 100.25,4.5 v100.48,4.72
  Bottom 0.406: 3V4.1 116.03,6.63 116.03,6.25 113.74,3.96 108.56,3.96 v107.95,4.57 107.87,4.72 v100.48,4.72 | v94.08,4.5 93.85,4.27 93.85,2.59 6103CAP9.1
VREF2_EN1  (via drill 0.61)
  Top 0.406: v107.95,82.04 107.95,81.36 106.73,80.14 S2.15 | v94.08,81.97 100.25,81.97 v100.48,82.19
  Bottom 0.406: 3V2.1 116.03,84.1 116.03,83.72 113.74,81.43 108.56,81.43 v107.95,82.04 107.87,82.19 v100.48,82.19 | v94.08,81.97 93.85,81.74 93.85,80.06 6103CAP3.1
VREF3
  Bottom 0.406: 125.78,49.53 125.78,19.81 126.54,19.05 132.03,19.05 138.74,12.34 138.74,7.85 136.91,6.02 3V5.2 | 125.78,49.53 127,50.75 SV4.20 | 125.78,49.53 125.63,49.61 124.48,50.75 SV4.18 124.26,50.83 122.05,50.83 SV4.16 121.89,50.83 119.53,50.83 SV4.14 119.38,50.83 117.02,50.83 SV4.12 116.79,50.83 114.43,50.83 SV4.10 114.28,50.83 111.91,50.83 SV4.8 111.76,50.83 109.4,50.83 SV4.6 109.17,50.83 106.81,50.83 SV4.4 106.66,50.83 104.29,50.83 SV4.2 104.14,50.75 102.92,49.53 102.92,23.09 93.85,14.02 6103CAP12.1
VREF3_EN  (via drill 0.61)
  Top 0.406: v135,9.45 v137.74,9.45 | v99.34,3.12 94.08,3.12 93.09,4.12 93.09,4.88 93.7,5.49 94.46,5.49 94.61,5.33 98.58,5.33 98.96,5.71 100.94,5.71 103.99,2.67 104.14,2.67 S1.14
  Bottom 0.406: v137.74,9.45 136.91,8.61 136.91,7.92 3V5.1 | 6103CAP11.1 134.54,11.43 135,10.97 v135,9.45 134.85,9.37 133.4,7.92 125.93,7.92 120.6,2.59 100.25,2.59 99.72,3.12 v99.34,3.12
VREF3_EN1  (via drill 0.61)
  Top 0.406: v135,86.92 v137.74,86.92 | v99.34,80.59 94.08,80.59 93.09,81.58 93.09,82.35 93.7,82.96 94.46,82.96 94.61,82.8 98.58,82.8 98.96,83.19 100.94,83.19 103.99,80.14 104.14,80.14 S2.14
  Bottom 0.406: v137.74,86.92 136.91,86.08 136.91,85.39 3V6.1 | 6103CAP5.1 134.54,88.9 135,88.44 v135,86.92 134.85,86.84 133.4,85.39 125.93,85.39 120.6,80.06 100.25,80.06 99.72,80.59 v99.34,80.59
VREF4  (via drill 0.61)
  Top 0.406: SV7.20 127,118.16 124.64,118.16 SV7.18 124.41,118.08 122.12,118.08 SV7.16 121.89,118.16 119.53,118.16 SV7.14 119.38,118.16 117.02,118.16 SV7.12 116.79,118.08 114.5,118.08 SV7.10 114.28,118.16 111.91,118.16 SV7.8 111.76,118.16 109.4,118.16 SV7.6 109.17,118.08 106.88,118.08 SV7.4 106.66,118.16 104.14,118.16 SV7.2 103.99,118.01 102.92,118.01 90.04,105.13 90.04,92.33 v97.89,84.48
  Bottom 0.406: 97.78,83.53 100.56,80.75 114.58,80.75 118.01,84.18 118.01,85.09 119.38,86.46 6103CAP2.1 | 97.78,83.53 97.66,83.64 96.22,83.64 3V1.2 | v97.89,84.48 97.89,83.64 97.78,83.53
VREF5
  Top 0.406: SV6.2 SV6.4 SV6.6 SV6.8 SV6.10 SV6.12 SV6.14 SV6.16 SV6.18 SV6.20
  Bottom 0.406: 3V2.2 114.12,84.18 112.83,84.18 110.54,86.46 6103CAP4.1 110.54,86.69 110.54,106.73 SV6.8
VREF6
  Bottom 0.406: 125.78,127 125.78,97.28 126.54,96.52 132.03,96.52 138.74,89.81 138.74,85.32 136.91,83.49 3V6.2 | 125.78,127 127,128.22 SV8.20 | 125.78,127 125.63,127.08 124.48,128.22 SV8.18 124.26,128.29 122.05,128.29 SV8.16 121.89,128.29 119.53,128.29 SV8.14 119.38,128.29 117.02,128.29 SV8.12 116.79,128.29 114.43,128.29 SV8.10 114.28,128.29 111.91,128.29 SV8.8 111.76,128.29 109.4,128.29 SV8.6 109.17,128.29 106.81,128.29 SV8.4 106.66,128.29 104.29,128.29 SV8.2 104.14,128.22 102.92,127 102.92,100.56 93.85,91.49 6103CAP6.1

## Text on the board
bNames: Solar Jackets Power Distribution Board / 12/7/2012 REV 4 | Solar Jackets Power Distribution Board / 12/7/2012 REV 4
tValues: Fan Control Board / 1-9-13 REV 1 | GND | 12V | - | OUTPUT | + | v7805 | 12V | GND | Pinout Header 1-3: / 1-19 ODD: GND / 2-20 EVEN: VREF | HEADER 1 | 1 | SOLAR JACKETS AIR GAP BOARD / 1/8/13 REV 4 | 2 | 12V | GND | 12V | GND | 3 | 4 | Pinout Header 4: / 1-19 ODD: GND / 2: 3.3V 3 / 4: 3.3V 2 / 6: 3.3V 1 / 8: 5V 3 / 10: 5V 2 / 12: 5V 1 / 14: 12V 2 / 16: 12V 1 / 18: 12V / 20: 12V | Fan Control Board / 1-9-13 REV 1 | Fan Control Board / 1-9-13 REV 1 | Switches: / 1: 12V 1 / 2: 12V 2 / 3: 5V 1 / 4: 5V 2 / 5: 5V 3 / 6: 3.3V 1 / 7: 3.3V 2 / 8: 3.3V 3 / 9: VREF 1 / 10: VREF 2 / 11: VREF 3 / 12: TS-7800 | - | GND | 12V | GND | 12V | + | v7805 | OUTPUT | OUTPUT | Pinout Header 1-3: / 1-19 ODD: GND / 2-20 EVEN: VREF | HEADER 1 | 12V | GND | 12V | GND | 1 | SOLAR JACKETS AIR GAP BOARD / 1/8/13 REV 4 | 2 | 3 | Fan Control Board / 1-9-13 REV 1 | Fan Control Board / 1-9-13 REV 1 | 4 | Pinout Header 4: / 1-19 ODD: GND / 2: 3.3V 3 / 4: 3.3V 2 / 6: 3.3V 1 / 8: 5V 3 / 10: 5V 2 / 12: 5V 1 / 14: 12V 2 / 16: 12V 1 / 18: 12V / 20: 12V | GND | 12V | GND | 12V | Switches: / 1: 12V 1 / 2: 12V 2 / 3: 5V 1 / 4: 5V 2 / 5: 5V 3 / 6: 3.3V 1 / 7: 3.3V 2 / 8: 3.3V 3 / 9: VREF 1 / 10: VREF 2 / 11: VREF 3 / 12: TS-7800 | OUTPUT | OUTPUT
